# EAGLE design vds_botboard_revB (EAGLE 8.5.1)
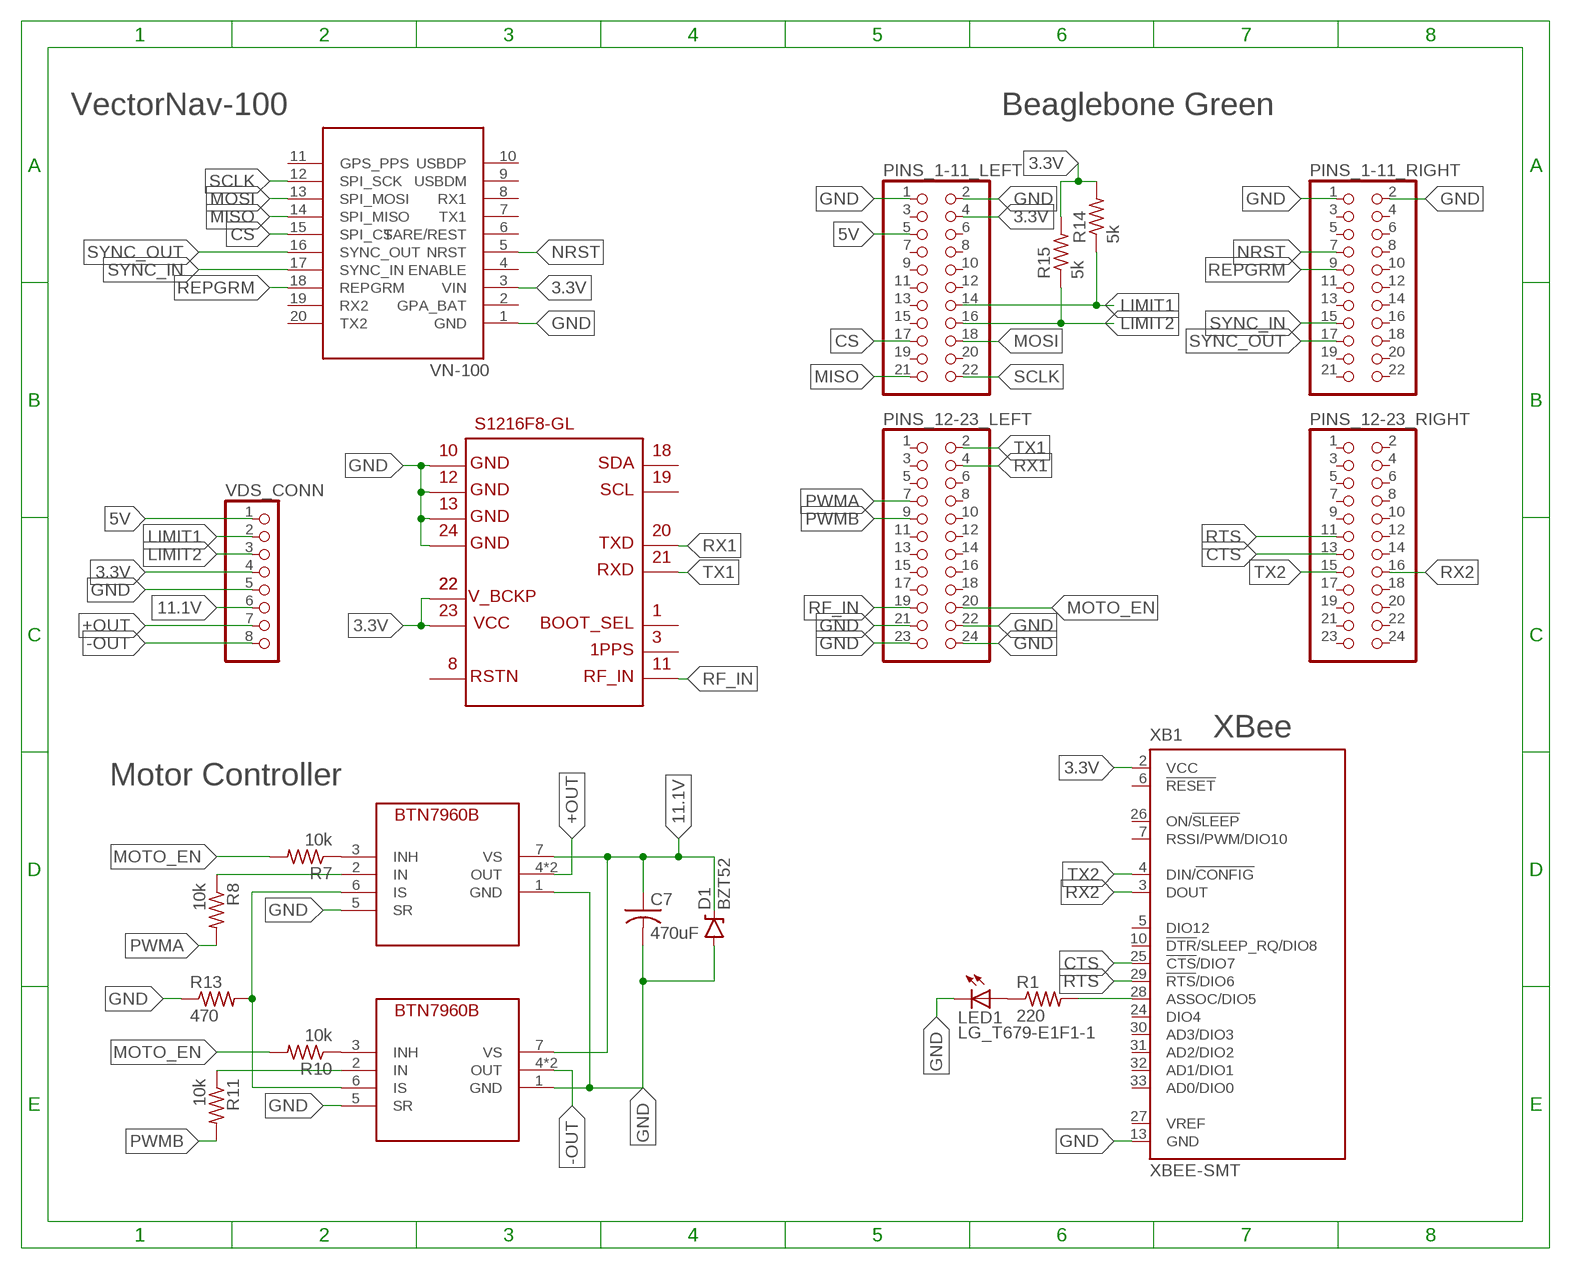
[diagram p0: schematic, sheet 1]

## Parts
C7  470uF  C-US050-024X044  [C050-024X044]
D1  BZT52  DIODE-ZENER  [DIODE-BZT52]
JM1  S1216F8-GL  [S1216F8-GL]
LED1  LG_T679-E1F1-1  [PLCC2]
PINS_1-11_LEFT  PINHD-2X11  [2X11]
PINS_1-11_RIGHT  PINHD-2X11  [2X11]
PINS_12-23_LEFT  PINHD-2X12  [2X12]
PINS_12-23_RIGHT  PINHD-2X12  [2X12]
R1  220  R-US_0204/5  [0204/5]
R7  10k  R-US_0204/5  [0204/5]
R8  10k  R-US_0204/5  [0204/5]
R10  10k  R-US_0204/5  [0204/5]
R11  10k  R-US_0204/5  [0204/5]
R13  470  R-US_0204/5  [0204/5]
R14  5k  R-US_0204/5  [0204/5]
R15  5k  R-US_0204/5  [0204/5]
U1  INF-PG-TO263-7-1_L_1_BTN7960B  [INF-PG-TO263-7-1_L_1PRIMARY]
U2  INF-PG-TO263-7-1_L_1_BTN7960B  [INF-PG-TO263-7-1_L_1PRIMARY]
VDS_CONN  PINHD-1X8  [1X08]
VN1  VECTORNAV-100  [VN-100]
XB1  XBEE-SMT  [XBEE-SMT]

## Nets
3.3V: JM1.22 JM1.23 PINS_1-11_LEFT.4 R14.2 R15.2 VDS_CONN.4 VN1.3(VIN) XB1.2(VCC)
5V: PINS_1-11_LEFT.5 VDS_CONN.1
11.1V: C7.1 D1.C U1.7(VS) U2.7(VS) VDS_CONN.6
+OUT: U1.4(OUT) U1.8(OUT) VDS_CONN.7
-OUT: U2.4(OUT) U2.8(OUT) VDS_CONN.8
COMM: R1.2 XB1.28(ASSOC/DIO5)
CS: PINS_1-11_LEFT.17 VN1.15(SPI_CS)
CTS: PINS_12-23_RIGHT.13 XB1.25(!CTS!/DIO7)
GND: C7.2 D1.A JM1.10 JM1.12 JM1.13 JM1.24 LED1.C PINS_1-11_LEFT.1 PINS_1-11_LEFT.2 PINS_1-11_RIGHT.1 PINS_1-11_RIGHT.2 PINS_12-23_LEFT.21 PINS_12-23_LEFT.22 PINS_12-23_LEFT.23 PINS_12-23_LEFT.24 R13.1 U1.1(GND) U1.5(SR) U2.1(GND) U2.5(SR) VDS_CONN.5 VN1.1(GND) XB1.13(GND)
IS: R13.2 U1.6(IS) U2.6(IS)
LIMIT1: PINS_1-11_LEFT.14 R14.1 VDS_CONN.2
LIMIT2: PINS_1-11_LEFT.16 R15.1 VDS_CONN.3
MISO: PINS_1-11_LEFT.21 VN1.14(SPI_MISO)
MOSI: PINS_1-11_LEFT.18 VN1.13(SPI_MOSI)
MOTO_EN: PINS_12-23_LEFT.20 R7.2 R10.2
N$1: LED1.A R1.1
N$7: R7.1 U1.3(INH)
N$8: R8.1 U1.2(IN)
N$9: R10.1 U2.3(INH)
N$10: R11.1 U2.2(IN)
NRST: PINS_1-11_RIGHT.7 VN1.5(NRST)
PWMA: PINS_12-23_LEFT.7 R8.2
PWMB: PINS_12-23_LEFT.9 R11.2
REPGRM: PINS_1-11_RIGHT.9 VN1.18(REPGRM)
RF_IN: JM1.11 PINS_12-23_LEFT.19
RTS: PINS_12-23_RIGHT.11 XB1.29(!RTS!/DIO6)
RX1: JM1.20 PINS_12-23_LEFT.4
RX2: PINS_12-23_RIGHT.16 XB1.3(DOUT)
SCLK: PINS_1-11_LEFT.22 VN1.12(SPI_SCK)
SYNC_IN: PINS_1-11_RIGHT.15 VN1.17(SYNC_IN)
SYNC_OUT: PINS_1-11_RIGHT.17 VN1.16(SYNC_OUT)
TX1: JM1.21 PINS_12-23_LEFT.2
TX2: PINS_12-23_RIGHT.15 XB1.4(DIN/!CONFIG)
Unconnected: JM1.1 JM1.3 JM1.8 JM1.18 JM1.19 PINS_1-11_LEFT.3 PINS_1-11_LEFT.6 PINS_1-11_LEFT.7 PINS_1-11_LEFT.8 PINS_1-11_LEFT.9 PINS_1-11_LEFT.10 PINS_1-11_LEFT.11 PINS_1-11_LEFT.12 PINS_1-11_LEFT.13 PINS_1-11_LEFT.15 PINS_1-11_LEFT.19 PINS_1-11_LEFT.20 PINS_1-11_RIGHT.3 PINS_1-11_RIGHT.4 PINS_1-11_RIGHT.5 PINS_1-11_RIGHT.6 PINS_1-11_RIGHT.8 PINS_1-11_RIGHT.10 PINS_1-11_RIGHT.11 PINS_1-11_RIGHT.12 PINS_1-11_RIGHT.13 PINS_1-11_RIGHT.14 PINS_1-11_RIGHT.16 PINS_1-11_RIGHT.18 PINS_1-11_RIGHT.19 PINS_1-11_RIGHT.20 PINS_1-11_RIGHT.21 PINS_1-11_RIGHT.22 PINS_12-23_LEFT.1 PINS_12-23_LEFT.3 PINS_12-23_LEFT.5 PINS_12-23_LEFT.6 PINS_12-23_LEFT.8 PINS_12-23_LEFT.10 PINS_12-23_LEFT.11 PINS_12-23_LEFT.12 PINS_12-23_LEFT.13 PINS_12-23_LEFT.14 PINS_12-23_LEFT.15 PINS_12-23_LEFT.16 PINS_12-23_LEFT.17 PINS_12-23_LEFT.18 PINS_12-23_RIGHT.1 PINS_12-23_RIGHT.2 PINS_12-23_RIGHT.3 PINS_12-23_RIGHT.4 PINS_12-23_RIGHT.5 PINS_12-23_RIGHT.6 PINS_12-23_RIGHT.7 PINS_12-23_RIGHT.8 PINS_12-23_RIGHT.9 PINS_12-23_RIGHT.10 PINS_12-23_RIGHT.12 PINS_12-23_RIGHT.14 PINS_12-23_RIGHT.17 PINS_12-23_RIGHT.18 PINS_12-23_RIGHT.19 PINS_12-23_RIGHT.20 PINS_12-23_RIGHT.21 PINS_12-23_RIGHT.22 PINS_12-23_RIGHT.23 PINS_12-23_RIGHT.24 VN1.2(GPA_BAT) VN1.4(ENABLE) VN1.6(TARE/REST) VN1.7(TX1) VN1.8(RX1) VN1.9(USBDM) VN1.10(USBDP) VN1.11(GPS_PPS) VN1.19(RX2) VN1.20(TX2) XB1.5(DIO12) XB1.6(!RESET) XB1.7(RSSI/PWM/DIO10) XB1.10(!DTR!/SLEEP_RQ/DIO8) XB1.24(DIO4) XB1.26(ON/!SLEEP) XB1.27(VREF) XB1.30(AD3/DIO3) XB1.31(AD2/DIO2) XB1.32(AD1/DIO1) XB1.33(AD0/DIO0)

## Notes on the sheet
- VectorNav-100 | Beaglebone Green
- XBee
- Motor Controller

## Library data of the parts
C7 = adafruit:C-US: CAPACITOR, American symbol
D1 = SparkFun-DiscreteSemi:DIODE-ZENER: Zener Diode; PROD-ID: DIO-08199
JM1 = S1216F8-GL:S1216F8-GL
LED1 = led:*_T679-?-1: LC TOPLED® Low Current LED; COLOR: green
PINS_1-11_LEFT PINS_1-11_RIGHT = pinhead:PINHD-2X11: PIN HEADER
PINS_12-23_LEFT PINS_12-23_RIGHT = pinhead:PINHD-2X12: PIN HEADER
R1 = resistor:R-US_: RESISTOR, American symbol
R7 R8 R10 R11 R13-R15 = adafruit:R-US_: RESISTOR, American symbol
U1 U2 = INF-PG-TO263-7-1L:INF-PG-TO263-7-1_L_1
VDS_CONN = pinhead:PINHD-1X8: PIN HEADER
VN1 = Vectornav-100_Breakout:VECTORNAV-100
XB1 = xbee:XBEE-SMT: XBee(TM)/XBee-PRO(TM) ZB SMT RF Modules. Source: Digi (90002002_a.pdf) (http://www.digi.com/products/wireless-wired-embedded-solutions/zigbee-rf-modules/zigbee-mesh-module/xbee-smt.jsp#overview)

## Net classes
0 default: width 1.016 mm, drill 0.508 mm, clearance 1.016 mm

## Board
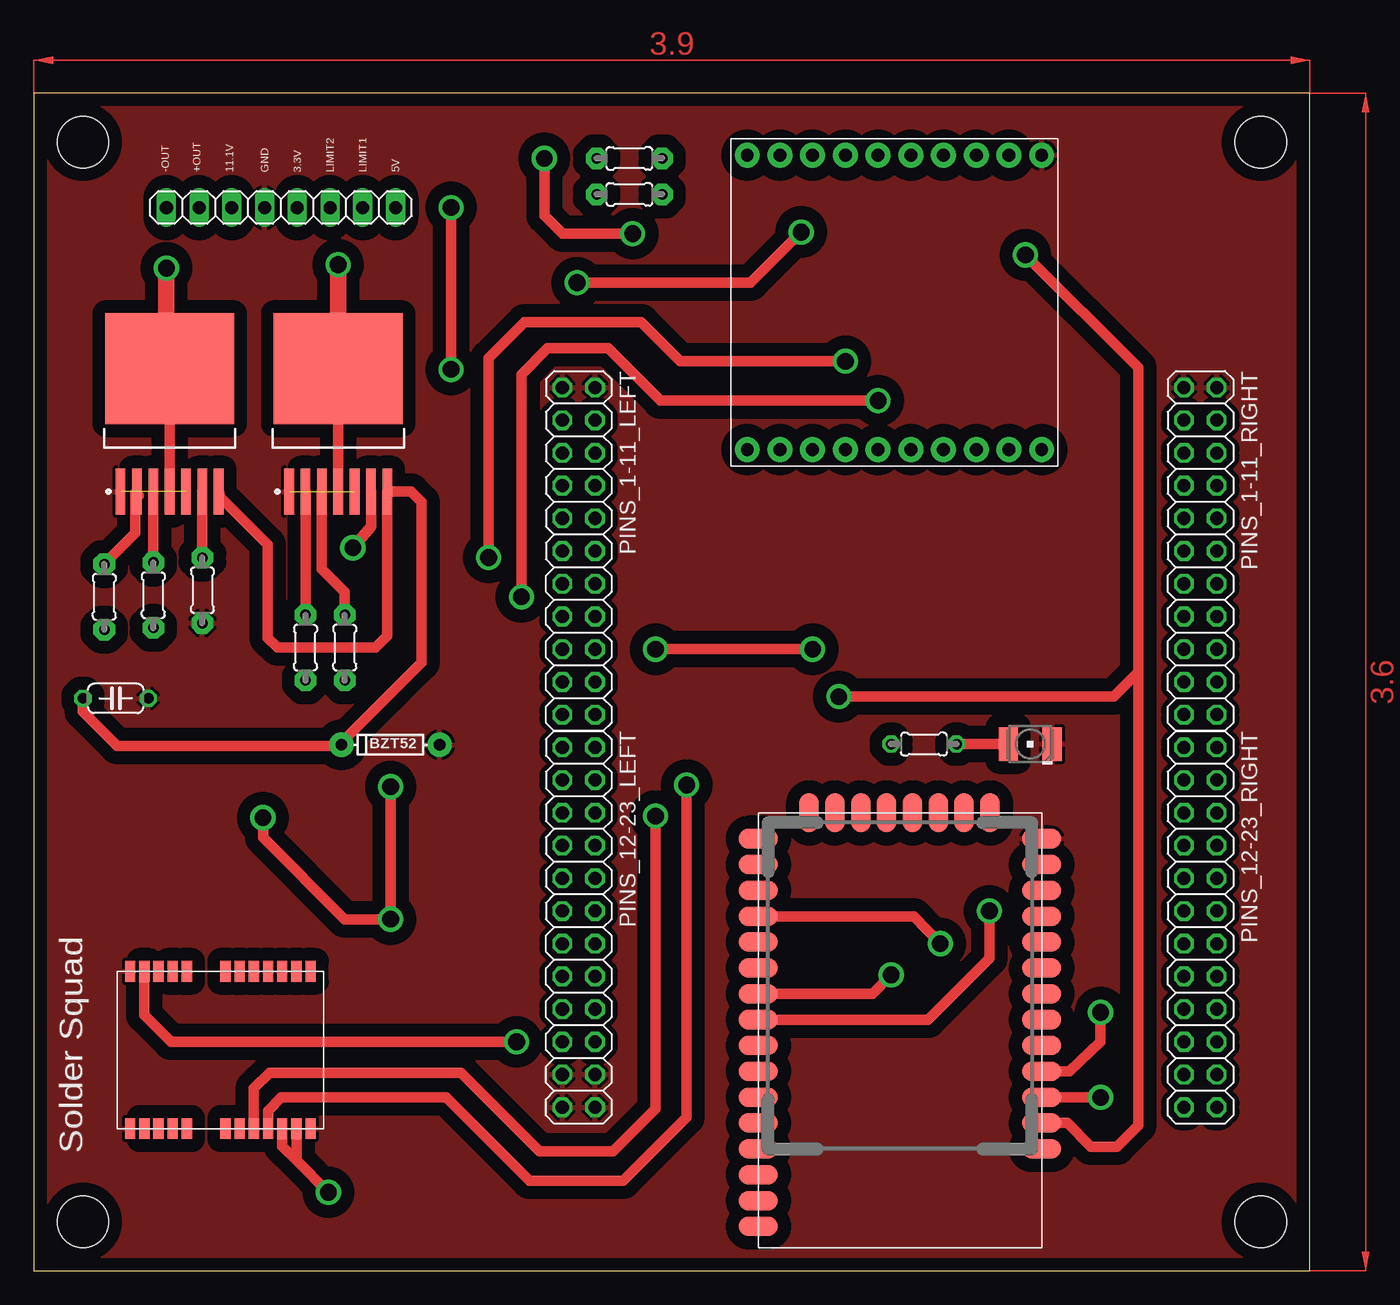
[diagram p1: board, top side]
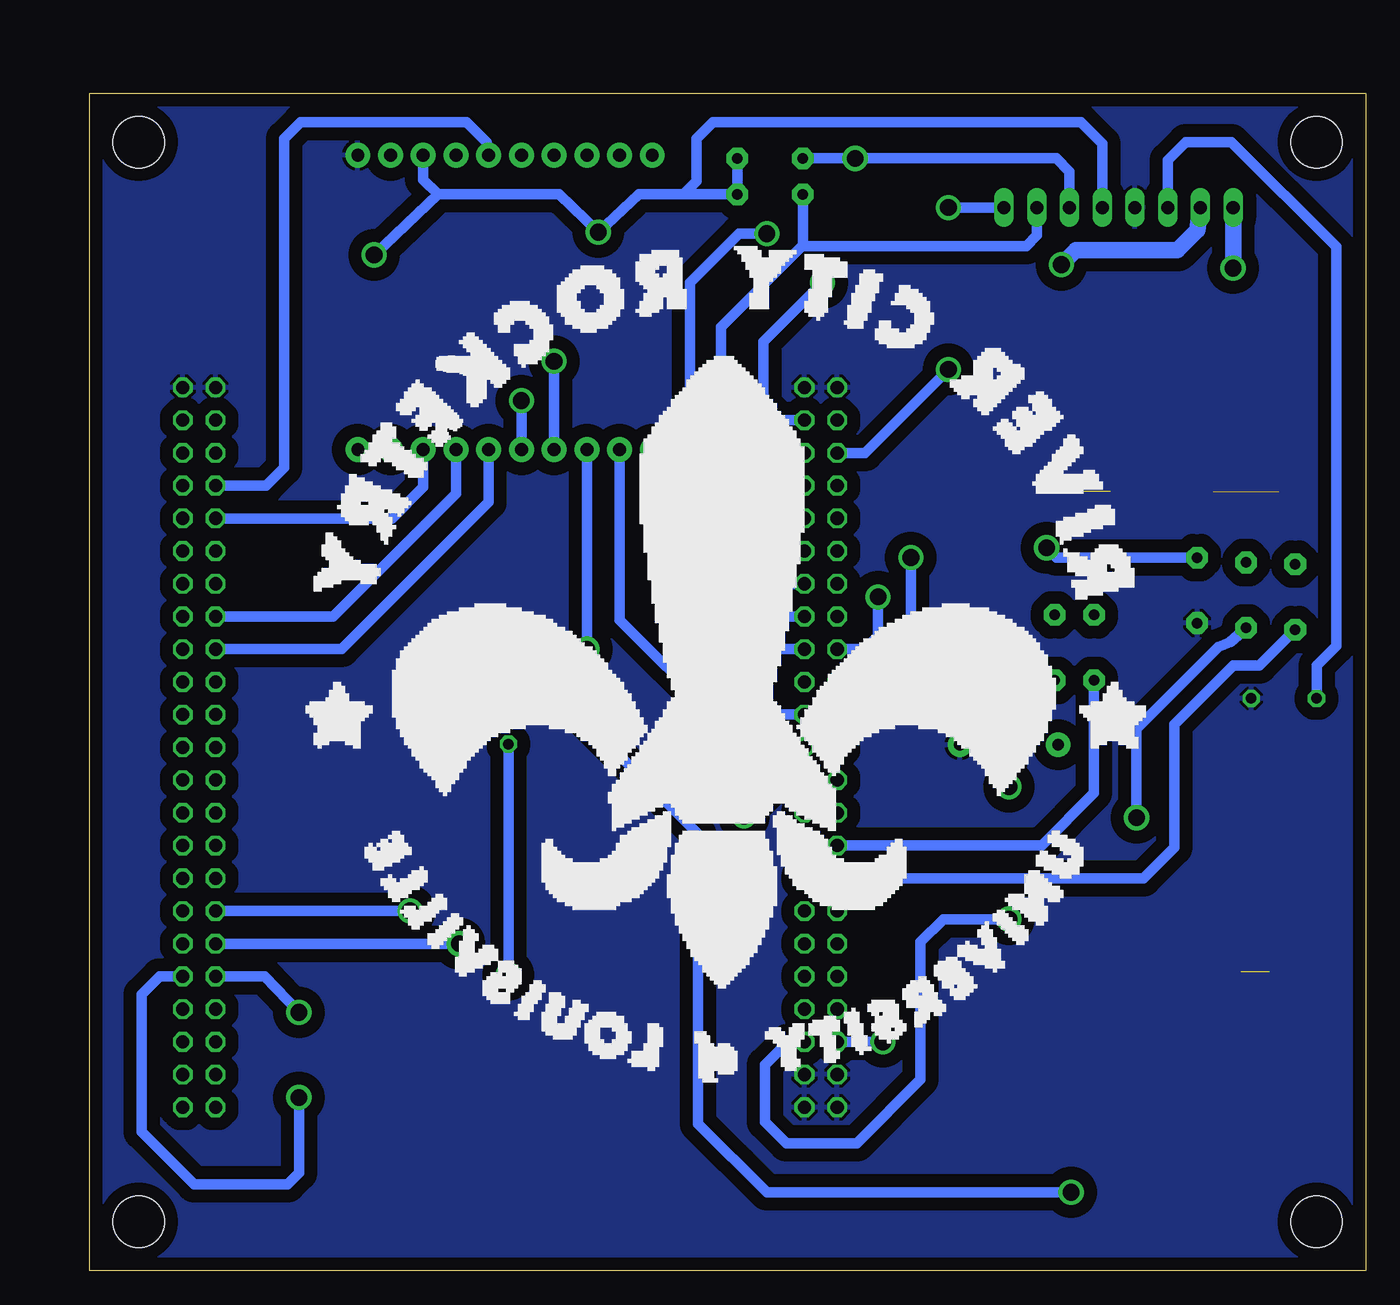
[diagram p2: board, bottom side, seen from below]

Size 99.06 x 91.44 mm. Coordinates in mm from the lower left corner, seen from the top.
Outline: 0,0 99.06,0 99.06,91.44 0,91.44 0,0
Copper layers (1*16): Top 0.035mm / dielectric 1.5mm / Bottom 0.035mm
Design rules "default *": minimum track width 10mil, minimum drill 50mil, track to track 10mil, track to pad 10mil, pad to pad 10mil, via to via 5mil, smd to smd 10mil, copper to edge 40mil, drill to drill 8mil, minimum pad ring 10mil, minimum via ring 8mil, stop-mask expansion 4mil, vias tented up to drill 0mil, thermal gap 10mil
Holes 4 mm at 3.81,87.63 95.25,87.63 3.81,3.81 95.25,3.81

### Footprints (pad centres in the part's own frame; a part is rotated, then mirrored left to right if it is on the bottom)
C050-024X044 = drill 0.813 octagon: 1 -2.54,0; 2 2.54,0
DIODE-BZT52 = drill 0.9 pad 1.88: A -3.81,0; C 3.81,0
S1216F8-GL = smd 1.6 x 0.8: 1 12.2,1; 2 12.2,2.1; 3 12.2,3.2; 4 12.2,4.3; 5 12.2,5.4; 6 12.2,6.5; 7 12.2,7.6; 8 12.2,10.6; 9 12.2,11.7; 10 12.2,12.8; 11 12.2,13.9; 12 12.2,15; 13 0,15; 14 0,13.9; 15 0,12.8; 16 0,11.7; 17 0,10.6; 18 0,7.6; 19 0,6.5; 20 0,5.4; 21 0,4.3; 22 0,3.2; 23 0,2.1; 24 0,1
PLCC2 = smd 2.6 x 1.5: A 0,1.7; C 0,-1.7
2X11 = drill 1.016 octagon: 1 -12.7,-1.27; 2 -12.7,1.27; 3 -10.16,-1.27; 4 -10.16,1.27; 5 -7.62,-1.27; 6 -7.62,1.27; 7 -5.08,-1.27; 8 -5.08,1.27; 9 -2.54,-1.27; 10 -2.54,1.27; 11 0,-1.27; 12 0,1.27; 13 2.54,-1.27; 14 2.54,1.27; 15 5.08,-1.27; 16 5.08,1.27; 17 7.62,-1.27; 18 7.62,1.27; 19 10.16,-1.27; 20 10.16,1.27; 21 12.7,-1.27; 22 12.7,1.27
2X12 = drill 1.016 octagon: 1 -13.97,-1.27; 2 -13.97,1.27; 3 -11.43,-1.27; 4 -11.43,1.27; 5 -8.89,-1.27; 6 -8.89,1.27; 7 -6.35,-1.27; 8 -6.35,1.27; 9 -3.81,-1.27; 10 -3.81,1.27; 11 -1.27,-1.27; 12 -1.27,1.27; 13 1.27,-1.27; 14 1.27,1.27; 15 3.81,-1.27; 16 3.81,1.27; 17 6.35,-1.27; 18 6.35,1.27; 19 8.89,-1.27; 20 8.89,1.27; 21 11.43,-1.27; 22 11.43,1.27; 23 13.97,-1.27; 24 13.97,1.27
0204/5 = drill 0.813 octagon: 1 -2.54,0; 2 2.54,0
0204/5' = drill 0.813 pad 1.676 octagon: 1 -2.54,0; 2 2.54,0
INF-PG-TO263-7-1_L_1PRIMARY = smd 3.55 x 0.75: 1 -6.05,3.81; 2 -6.05,2.54; 3 -6.05,1.27; 4 -6.05,0; 5 -6.05,-1.27; 6 -6.05,-2.54; 7 -6.05,-3.81 | smd 8.6 x 10: 8 3.5,0
1X08 = drill 1.016 long: 1 -8.89,0; 2 -6.35,0; 3 -3.81,0; 4 -1.27,0; 5 1.27,0; 6 3.81,0; 7 6.35,0; 8 8.89,0
VN-100 = drill 1 pad 1.93: 1 24.13,1.27; 2 24.13,3.81; 3 24.13,6.35; 4 24.13,8.89; 5 24.13,11.43; 6 24.13,13.97; 7 24.13,16.51; 8 24.13,19.05; 9 24.13,21.59; 10 24.13,24.13; 11 1.27,24.13; 12 1.27,21.59; 13 1.27,19.05; 14 1.27,16.51; 15 1.27,13.97; 16 1.27,11.43; 17 1.27,8.89; 18 1.27,6.35; 19 1.27,3.81; 20 1.27,1.27
XBEE-SMT = smd 3.048 x 1.524: 1 0,26.086; 2 0,24.079; 3 0,22.073; 4 0,20.066; 5 0,18.059; 6 0,16.053; 7 0,14.046; 8 0,12.04; 9 0,10.033; 10 0,8.026; 11 0,6.02; 12 0,4.013; 13 0,2.007; 22 21.996,2.007; 23 21.996,4.013; 24 21.996,6.02; 25 21.996,8.026; 26 21.996,10.033; 27 21.996,12.04; 28 21.996,14.046; 29 21.996,16.053; 30 21.996,18.059; 31 21.996,20.066; 32 21.996,22.073; 33 21.996,24.079; 34 21.996,26.086; 35 21.996,28.092; 36 21.996,30.099; 37 21.996,32.106 | smd 1.524 x 3.048: 14 4.013,0; 15 6.02,0; 16 8.026,0; 17 10.033,0; 18 12.04,0; 19 14.046,0; 20 16.053,0; 21 18.059,0

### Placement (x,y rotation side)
C7  6.35,44.45 0 top
D1  27.69,40.84 180 top
JM1  22.48,11.05 90 top
LED1  77.34,40.89 90 top
PINS_1-11_LEFT  42.29,55.88 270 top
PINS_1-11_RIGHT  90.55,55.88 270 top
PINS_12-23_LEFT  42.29,26.67 270 top
PINS_12-23_RIGHT  90.55,26.67 270 top
R1  69.09,40.89 180 top
R7  10k  [0204/5']  24.13,48.39 270 top
R8  10k  [0204/5']  21.08,48.39 270 top
R10  10k  [0204/5']  9.27,52.45 270 top
R11  10k  [0204/5']  5.46,52.32 270 top
R13  470  [0204/5']  13.08,52.83 90 top
R14  5k  [0204/5']  46.23,83.57 0 top
R15  5k  [0204/5']  46.23,86.36 0 top
U1  23.62,66.55 90 top
U2  10.54,66.55 90 top
VDS_CONN  19.18,82.55 180 top
VN1  79.5,62.48 90 top
XB1  78.23,35.56 180 top

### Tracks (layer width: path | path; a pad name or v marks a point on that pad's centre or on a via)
3.3V  (via drill 1.3 pad 1.95)
  Top 0.813: XB1.2 80.21,11.48 82.04,9.65 84.07,9.65 85.72,11.3 85.72,46.48 | 20.38,8.58 JM1.23 | 20.38,8.58 v22.86,6.1 | JM1.22 19.28,9.68 20.38,8.58 | v42.16,76.71 55.63,76.71 v59.56,80.64 | v62.48,44.58 83.82,44.58 85.72,46.48 | v76.96,78.87 85.72,70.1 85.72,46.48
  Bottom 0.813: R15.2 R14.2 52.96,83.57 | 52.96,83.57 56.39,83.57 v59.56,80.64 62.61,83.57 72.01,83.57 | 72.01,83.57 73.15,84.71 VN1.3 | 72.01,83.57 v76.96,78.87 | VDS_CONN.4 20.45,87.5 22.1,89.15 50.67,89.15 51.94,87.88 51.94,84.58 52.96,83.57 | v22.86,6.1 46.48,6.1 51.82,11.43 51.82,33.91 v62.48,44.58 | PINS_1-11_LEFT.4 45.47,66.04 46.74,67.31 46.74,72.14 v42.16,76.71
5V  (via drill 1.3 pad 1.95)
  Top 0.813: v32.38,82.55 v32.38,69.98
  Bottom 0.813: v32.38,69.98 38.86,63.5 PINS_1-11_LEFT.5 | VDS_CONN.1 v32.38,82.55
11.1V
  Top 0.813: 27.45,60.52 U1.7 | U2.7 14.48,60.07 18.16,56.39 18.16,49.15 18.92,48.39 26.54,48.39 27.43,49.28 U1.7 | U1.7 29.29,60.5 30.1,59.69 30.1,47.24 23.88,41.02 D1.C 23.8,40.77 6.48,40.77 3.81,43.43 C7.1
  Bottom 0.813: 23.8,40.77 D1.C | C7.1 3.81,46.99 2.29,48.51 2.29,79.5 10.41,87.63 13.97,87.63 15.37,86.23 VDS_CONN.6
+OUT  (via drill 1.3 pad 1.95)
  Top 0.813: U1.8 U1.4
  Top 1.27: v23.62,78.11 U1.8
  Bottom 1.27: v23.62,78.11 22.48,79.25 14.61,79.25 13.08,80.77 VDS_CONN.7
-OUT  (via drill 1.3 pad 1.95)
  Top 0.813: U2.8 U2.4
  Top 1.27: v10.29,77.85 10.29,73.91 U2.8
  Bottom 1.27: v10.29,77.85 VDS_CONN.8
COMM  (via drill 1.3 pad 1.95)
  Top 0.813: XB1.28 65.08,21.51 v66.55,22.99
  Bottom 0.813: v66.55,22.99 R1.2
CS  (via drill 1.3 pad 1.95)
  Top 0.813: v37.85,52.32 37.85,69.6 39.88,71.63 44.58,71.63 48.64,67.56 v65.53,67.56
  Bottom 0.813: VN1.15 v65.53,67.56 | v37.85,52.32 37.85,49.28 38.86,48.26 PINS_1-11_LEFT.17
CTS  (via drill 1.3 pad 1.95)
  Top 0.813: XB1.25 68.3,27.53 v70.36,25.4
  Bottom 0.813: v70.36,25.4 PINS_12-23_RIGHT.13
GND  (3 unrouted)
  pour Top: 0,91.44 0,0 99.06,0 99.06,91.44
  pour Bottom: 0,91.44 0,0 99.06,0 99.06,91.44
  pour Top: 0,91.44 99.31,91.44 99.31,0 0,0
  pour Bottom: 0,91.31 99.19,91.31 99.19,0 0,0
IS  (via drill 1.3 pad 1.95)
  Top 0.813: U1.6 26.16,57.78 v24.77,56.13 | U2.6 R13.2
  Bottom 0.813: R13.2 24,55.37 v24.77,56.13
LIMIT1
  Bottom 0.813: R14.1 43.69,79.63 43.75,79.57 | PINS_1-11_LEFT.14 44.7,53.34 45.47,54.1 49.4,54.1 50.04,54.74 50.04,73.28 43.75,79.57 | VDS_CONN.2 25.53,80.39 26.35,79.57 43.75,79.57
LIMIT2  (via drill 1.3 pad 1.95)
  Top 0.813: v46.48,80.52 41.02,80.52 39.62,81.92 v39.62,86.36
  Bottom 0.813: PINS_1-11_LEFT.16 45.59,50.8 46.86,52.07 51.56,52.07 52.45,52.96 52.45,76.71 48.64,80.52 v46.48,80.52 | VDS_CONN.3 22.99,85.34 24,86.36 v39.62,86.36 R15.1
MISO  (via drill 1.3 pad 1.95)
  Top 0.813: v35.31,55.37 35.31,70.87 38.1,73.66 47.12,73.66 50.16,70.61 v62.99,70.61
  Bottom 0.813: VN1.14 v62.99,70.61 | PINS_1-11_LEFT.21 39.12,43.18 35.31,46.99 v35.31,55.37
MOSI  (via drill 1.3 pad 1.95)
  Top 0.813: v60.45,48.26 v48.26,48.26
  Bottom 0.813: VN1.13 v60.45,48.26 | v48.26,48.26 PINS_1-11_LEFT.18
MOTO_EN  (via drill 1.3 pad 1.95)
  Top 0.813: v17.78,35.18 17.78,33.66 24.13,27.3 v27.69,27.3 v27.69,37.59
  Bottom 0.813: v17.78,35.18 17.78,42.08 11.43,48.44 10.49,48.82 R10.2 | R7.2 27.69,42.29 v27.69,37.59 | v27.69,27.3 32.77,27.3 34.54,25.53 34.54,14.86 39.5,9.91 44.96,9.91 46.61,11.56 46.61,16 44.83,17.78 PINS_12-23_LEFT.20
N$1
  Top 0.813: R1.1 LED1.A
N$7
  Top 0.813: U1.3 22.35,54.48 24.13,52.7 R7.1
N$8
  Top 0.813: U1.2 R8.1
N$9
  Top 0.813: U2.3 R10.1
N$10
  Top 0.152: U2.2 7.87,60.37
  Top 0.813: U2.2 8.13,60.2 | 7.87,60.37 7.87,57.28 R11.1
NRST
  Bottom 0.813: VN1.5 68.22,86.77 68.22,87.6 69.78,89.15 82.68,89.15 83.95,87.88 83.95,62.36 85.34,60.96 PINS_1-11_RIGHT.7
PWMA
  Bottom 0.813: PINS_12-23_LEFT.7 25.15,33.02 21.08,37.08 R8.2
PWMB
  Bottom 0.813: PINS_12-23_LEFT.9 17.27,30.48 14.86,32.89 14.86,42.42 10.29,46.99 8.26,46.99 R11.2
REPGRM
  Bottom 0.813: VN1.18 73.15,60.83 75.56,58.42 PINS_1-11_RIGHT.9
RF_IN  (via drill 1.3 pad 1.95)
  Top 0.813: JM1.11 8.58,19.87 10.67,17.78 v37.47,17.78
  Bottom 0.813: v37.47,17.78 PINS_12-23_LEFT.19
RTS  (via drill 1.3 pad 1.95)
  Top 0.813: XB1.29 69.42,19.51 74.17,24.26 v74.17,27.94
  Bottom 0.813: v74.17,27.94 PINS_12-23_RIGHT.11
RX1  (via drill 1.3 pad 1.95)
  Top 0.813: JM1.20 17.08,14.16 18.29,15.37 33.15,15.37 39.24,9.27 44.96,9.27 48.26,12.57 v48.26,35.31
  Bottom 0.813: v48.26,35.31 45.47,38.1 PINS_12-23_LEFT.4
RX2  (via drill 1.3 pad 1.95)
  Top 0.813: XB1.3 78.77,13.46 v82.8,13.46
  Bottom 0.813: PINS_12-23_RIGHT.16 93.6,22.86 95,21.46 95,10.79 90.93,6.73 83.69,6.73 82.8,7.62 v82.8,13.46
SCLK
  Bottom 0.813: VN1.12 57.91,50.55 50.55,43.18 PINS_1-11_LEFT.22
SYNC_IN
  Bottom 0.813: VN1.17 70.61,60.33 80.14,50.8 PINS_1-11_RIGHT.15
SYNC_OUT
  Bottom 0.813: VN1.16 68.07,59.69 79.5,48.26 PINS_1-11_RIGHT.17
TX1  (via drill 1.3 pad 1.95)
  Top 0.813: v50.67,37.72 50.67,11.94 45.72,6.99 38.48,6.99 32,13.46 19.18,13.46 18.18,12.43 JM1.21
  Bottom 0.813: v50.67,37.72 50.67,38.99 49.02,40.64 PINS_12-23_LEFT.2
TX2  (via drill 1.3 pad 1.95)
  Top 0.813: XB1.4 80.39,15.49 82.8,17.78 v82.8,20.07
  Bottom 0.813: v82.8,20.07 85.47,22.86 PINS_12-23_RIGHT.15
(copper drawn outside any net)
  shapes: Top area x2

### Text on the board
tPlace: -OUT | +OUT | 11.1V | GND | 3.3V | LIMIT2 | LIMIT1 | 5V | Solder Squad

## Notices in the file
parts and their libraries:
SparkFun-DiscreteSemi: Licensing: Creative Commons ShareAlike 4.0 International - https://creativecommons.org/licenses/by-sa/4.0
